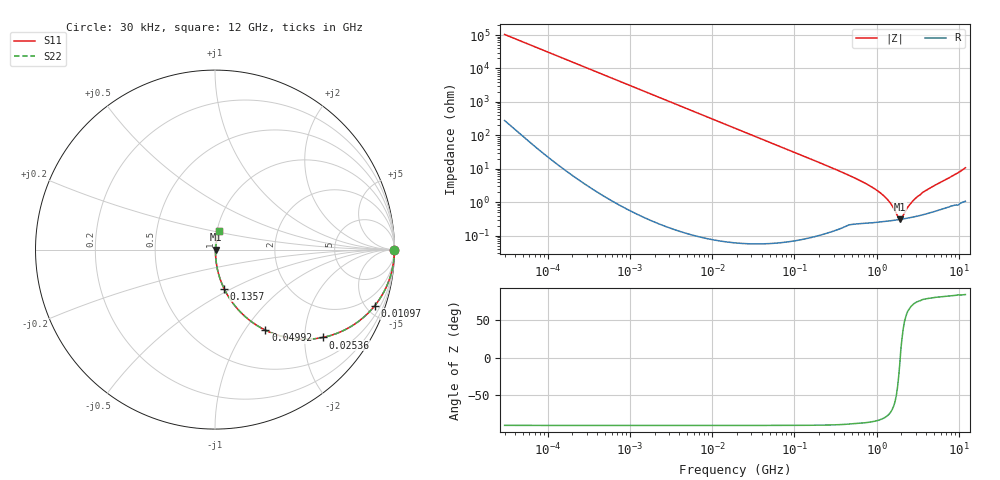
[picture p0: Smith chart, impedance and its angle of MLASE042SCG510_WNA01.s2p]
! MLASE042SCG510_WNA01  S-PARAMETER MODEL  ( General Type )
! Model Generated by TAIYO YUDEN Corporation (http://www.ty-top.com)
! Version 3.0
! TAIYO YUDEN Control No. 140604
! Copyright(c) 2013 TAIYO YUDEN CO.,LTD. All Rights Reserved.
! Product Description (link to TY-COMPAS)
! https://ds.yuden.co.jp/TYCOMPAS/or/detail?pn=MLASE042SCG510JWNA01&u=M
! Products Name : Multilayer Ceramic Capacitors
! Characteristics :
!  Capacitance : 51 pF , Rated Voltage : 16V , TCC : CG / C0G
!  Case Size : 0.4 x 0.2 / 0.016 x 0.008 [mm/inch] , Thickness : 0.2 / 0.008 [mm/inch]
!  (Conditions: Temperature = 25 degC , DC Bias Current/Voltage = 0A / 0V)
! External Node Assignments :
!  1  o---| |---o  2
! GND o---------o GND
! Frequency Range : 0.03MHz  -  12000MHz  [ 401 STEP ]
# MHz S RI R 50
! Freq[MHz].  S11 Real  S11 Imag  S21 Real  S21 Imag  S12 Real  S12 Imag  S22 Real  S22 Imag
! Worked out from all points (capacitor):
!   401 points, 30 kHz to 12 GHz, reference 50 ohm
!   read as one part in series: C = 51 pF near 32 kHz
!   lowest |Z| = 309 mohm at 1.909 GHz (marker M1)
!   series resonance near 1.936 GHz, so ESL is about 130 pH
!   S11 on the Smith chart (normalised r, x): 30 kHz: open; 10.97 MHz: 1.00, -5.69; 25.36 MHz: 1.00, -2.46; 49.92 MHz: 1.00, -1.25; 135.7 MHz: 1.00, -0.46; 12 GHz: 1.02, +0.21
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0.03  1 -0.000961  3.49e-06 0.000961  3.49e-06 0.000961  1 -0.000961
0.260295  0.9999 -0.00834  7.24e-05 0.00834  7.24e-05 0.00834  0.9999 -0.00834
2.258455  0.9948 -0.072  0.00522 0.072  0.00522 0.072  0.9948 -0.072
5.223303  0.9727 -0.1628  0.0273 0.1628  0.0273 0.1628  0.9727 -0.1628
10.96639  0.89 -0.3127  0.11 0.3127  0.11 0.3127  0.89 -0.3127
18.97367  0.73 -0.4438  0.27 0.4438  0.27 0.4438  0.73 -0.4438
25.36282  0.6021 -0.4892  0.3979 0.4892  0.3979 0.4892  0.6021 -0.4892
35.01459  0.4426 -0.4964  0.5574 0.4964  0.5574 0.4964  0.4426 -0.4964
49.92358  0.2809 -0.449  0.7191 0.449  0.7191 0.449  0.2809 -0.449
78.41115  0.1368 -0.3428  0.8632 0.3428  0.8632 0.3428  0.1368 -0.3428
135.6642  0.0505 -0.2172  0.9495 0.2172  0.9495 0.2172  0.0505 -0.2172
164.6252  0.035 -0.1814  0.965 0.1814  0.965 0.1814  0.035 -0.1814
749.4426  0.00359 -0.0352  0.9964 0.0352  0.9964 0.0352  0.00359 -0.0352
1103.571  0.00293 -0.019  0.9971 0.019  0.9971 0.019  0.00293 -0.019
1428.372  0.00285 -0.0099  0.9971 0.0099  0.9971 0.0099  0.00285 -0.0099
1790.1  0.00298 -0.00251  0.997 0.00251  0.997 0.00251  0.00298 -0.00251
1909.359  0.00304 -0.000474  0.997 0.000474  0.997 0.000474  0.00304 -0.000474
2036.564  0.00312 0.00152  0.9969 -0.00152  0.9969 -0.00152  0.00312 0.00152
2392.896  0.00338 0.0063  0.9966 -0.0063  0.9966 -0.0063  0.00338 0.0063
2722.352  0.00365 0.00989  0.9963 -0.00989  0.9963 -0.00989  0.00365 0.00989
3523.591  0.00442 0.0177  0.9956 -0.0177  0.9956 -0.0177  0.00442 0.0177
12000  0.0215 0.1033  0.9785 -0.1033  0.9785 -0.1033  0.0215 0.1033
